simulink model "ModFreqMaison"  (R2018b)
settings: Solver=FixedStepAuto  StartTime=0.0  StopTime=10  FixedStep=1e-5  RelTol=1e-4
libraries: simulink x1, commsynccomp2 x1, commrandsrc2 x1

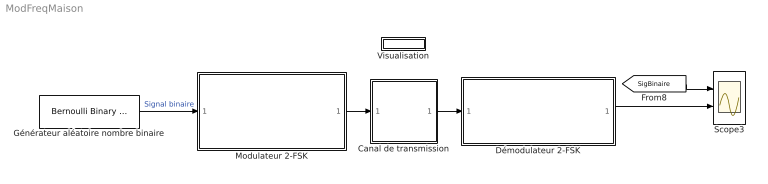
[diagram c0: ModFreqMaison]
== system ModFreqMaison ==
  Canal de transmission : Subsystem
  Démodulateur 2-FSK : Subsystem
  Générateur aléatoire nombre binaire : commrandsrc2/Bernoulli Binary Generator  P=0.4  seed=67  Ts=1  frameBased=off  sampPerFrame=1  orient=off  outDataType=double
  Modulateur 2-FSK : Subsystem
  Scope3 : Scope  NumInputPorts=2
  Visualisation : Subsystem
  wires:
  [SigBinaire] -> Scope3/1
  Générateur aléatoire nombre binaire/1 -> Modulateur 2-FSK/1(Signal binaire)  "Signal binaire"
  Modulateur 2-FSK/1(Signal Modulé FSK) -> Canal de transmission/1(In1)
  Démodulateur 2-FSK/1(Signal démodulé) -> Scope3/2
  Canal de transmission/1(Out1) -> Démodulateur 2-FSK/1(Signal modulé reçu)

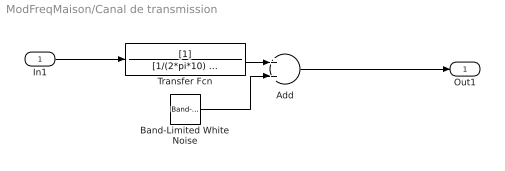
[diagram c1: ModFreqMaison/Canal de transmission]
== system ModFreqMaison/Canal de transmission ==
  In1 : Inport
  Add : Sum
  Band-Limited White Noise : simulink/Sources/Band-Limited White Noise  Cov=[0.002]  Ts=1  seed=[23341]
  Transfer Fcn : TransferFcn  Denominator=[1/(2*pi*10) 1]
  Out1 : Outport
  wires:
  Add/1 -> Out1/1
  Band-Limited White Noise/1 -> Add/2
  Transfer Fcn/1 -> Add/1
  In1/1 -> Transfer Fcn/1

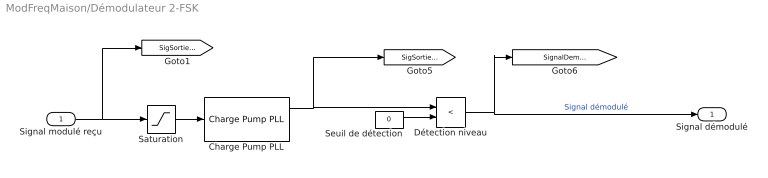
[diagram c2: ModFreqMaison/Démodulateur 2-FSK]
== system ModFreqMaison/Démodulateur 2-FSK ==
  Signal modulé reçu : Inport
  Charge Pump PLL : commsynccomp2/Charge Pump PLL  Fn=[2*pi*1]  Fd="[1   2*pi*1]"  Kvco=4  Fc=10  Ph=0  Ac=1
  Détection niveau : RelationalOperator  Operator=<  OutDataTypeStr=boolean
  Saturation : Saturate
  Seuil de détection : Constant  Value=0
  Signal démodulé : Outport
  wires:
  Charge Pump PLL/1 -> Détection niveau/1, [SigSortiePLL]
  Seuil de détection/1 -> Détection niveau/2
  Détection niveau/1 -> Signal démodulé/1, [SignalDemodule]  "Signal démodulé"
  Saturation/1 -> Charge Pump PLL/1
  Signal modulé reçu/1 -> [SigSortieCanal], Saturation/1

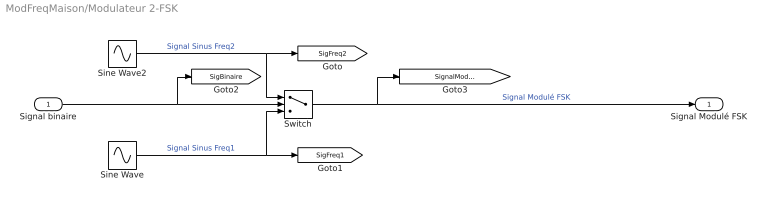
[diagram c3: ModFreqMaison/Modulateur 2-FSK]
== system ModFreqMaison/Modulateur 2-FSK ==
  Signal binaire : Inport
  Sine Wave : Sin  Frequency=2*pi*15  Samples=25  SampleTime=0.001
  Sine Wave2 : Sin  Frequency=2*pi*5  Samples=50  SampleTime=0.001
  Switch : Switch  Threshold=0.5
  Signal Modulé FSK : Outport
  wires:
  Sine Wave2/1 -> [SigFreq2], Switch/1  "Signal Sinus Freq2"
  Switch/1 -> Signal Modulé FSK/1, [SignalModuleFSK]  "Signal Modulé FSK"
  Sine Wave/1 -> Switch/3, [SigFreq1]  "Signal Sinus Freq1"
  Signal binaire/1 -> [SigBinaire], Switch/2

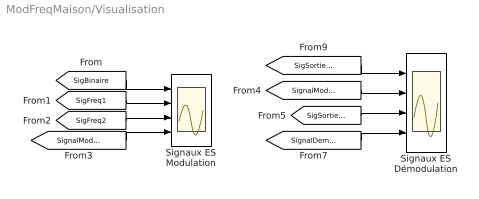
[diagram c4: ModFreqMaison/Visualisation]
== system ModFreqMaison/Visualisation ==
  Signaux ES Démodulation : Scope  NumInputPorts=4
  Signaux ES Modulation : Scope  NumInputPorts=4
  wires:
  [SignalModuleFSK] -> Signaux ES Démodulation/2
  [SignalModuleFSK] -> Signaux ES Modulation/4
  [SigFreq2] -> Signaux ES Modulation/3
  [SigFreq1] -> Signaux ES Modulation/2
  [SigBinaire] -> Signaux ES Modulation/1
  [SignalDemodule] -> Signaux ES Démodulation/4
  [SigSortiePLL] -> Signaux ES Démodulation/3
  [SigSortieCanal] -> Signaux ES Démodulation/1
